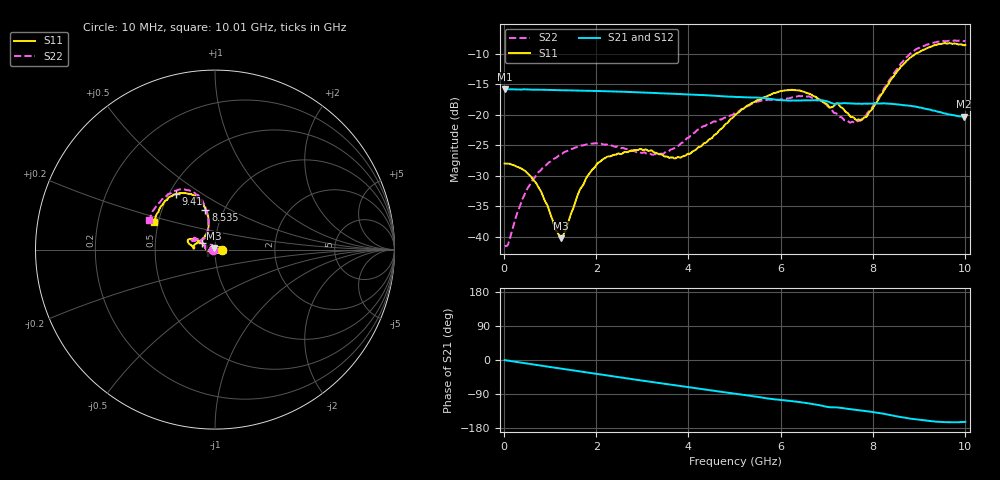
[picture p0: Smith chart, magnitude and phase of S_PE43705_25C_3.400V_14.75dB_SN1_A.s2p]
! Device ID: PE43705
! Serial: 1
! Insertion: A
! Impedance: 50 ohm
! Temp: 25C
! VDD: 3.400V
! Attenuation Step: 14.75dB
#  Hz  S  RI  R  50
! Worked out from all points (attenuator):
!   401 points, 10 MHz to 10.01 GHz, reference 50 ohm
!   highest |S21| = -15.77 dB at 10 MHz (marker M1); lowest = -20.3 dB at 9.985 GHz (marker M2)
!   lowest |S11| = -40.2 dB at 1.235 GHz (marker M3), VSWR 1.02, Z = 49.6 + j0.87 ohm
!   |S11| at or under -10 dB: start of sweep to 8.922 GHz
!   |S22| runs from -41.6 to -7.8 dB; largest |S21 - S12| = 0.0014
!   S11 on the Smith chart (normalised r, x): 10 MHz: 1.08, +0.00; 4.81 GHz: 0.86, +0.07; 8.535 GHz: 0.82, +0.39; 9.41 GHz: 0.54, +0.39; 10.01 GHz: 0.47, +0.17
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1e7  0.0399 0.000105  0.1628 -0.000706  0.1631 -0.000648  -0.0084 0.000516
1.1e8  0.0397 0.00252  0.1623 -0.00606  0.1622 -0.00602  -0.00764 0.00524
4.35e8  0.0332 0.0112  0.1605 -0.0232  0.16 -0.0228  -0.0113 0.0186
6.35e8  0.0254 0.0145  0.1578 -0.033  0.1577 -0.033  -0.0171 0.0244
1.235e9  -0.00421 0.00877  0.1472 -0.0615  0.1473 -0.0615  -0.0387 0.0274
1.685e9  -0.0252 -0.00493  0.1359 -0.081  0.1359 -0.0809  -0.0522 0.0207
2.21e9  -0.0377 -0.024  0.1194 -0.1011  0.1194 -0.1009  -0.0562 0.00996
2.935e9  -0.0401 -0.0334  0.0918 -0.1229  0.092 -0.1229  -0.0487 0.00938
3.36e9  -0.0381 -0.0284  0.0738 -0.1315  0.074 -0.1314  -0.0457 0.0123
3.885e9  -0.0454 -0.00655  0.051 -0.1387  0.0512 -0.1386  -0.0539 0.025
4.81e9  -0.0752 0.0382  0.0109 -0.1414  0.0111 -0.1413  -0.0809 0.0493
5.01e9  -0.0874 0.0477  0.00271 -0.1406  0.00296 -0.1407  -0.0889 0.0541
5.985e9  -0.1454 0.058  -0.0346 -0.1277  -0.0341 -0.1278  -0.1186 0.0616
6.685e9  -0.142 0.0302  -0.058 -0.1185  -0.058 -0.1185  -0.1281 0.0514
7.635e9  -0.0723 0.0553  -0.0821 -0.0924  -0.0819 -0.0925  -0.0547 0.067
7.885e9  -0.0478 0.0866  -0.0882 -0.0868  -0.0879 -0.0873  -0.0425 0.0948
8.36e9  -0.0374 0.1821  -0.1012 -0.0713  -0.1008 -0.0715  -0.0407 0.1891
8.535e9  -0.053 0.2233  -0.1041 -0.0628  -0.1037 -0.064  -0.0542 0.2341
8.935e9  -0.108 0.2999  -0.1074 -0.0465  -0.107 -0.0457  -0.1233 0.3224
9.41e9  -0.22 0.3096  -0.1015 -0.0313  -0.1016 -0.031  -0.2316 0.3263
9.985e9  -0.3337 0.165  -0.0928 -0.0277  -0.0929 -0.0276  -0.3626 0.1765
1.001e10  -0.3411 0.1564  -0.0928 -0.028  -0.0932 -0.0281  -0.3703 0.1654
